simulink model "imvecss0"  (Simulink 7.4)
settings: Solver=ode45  StartTime=0  StopTime=20  MaxStep=5e-4  RelTol=1e-3

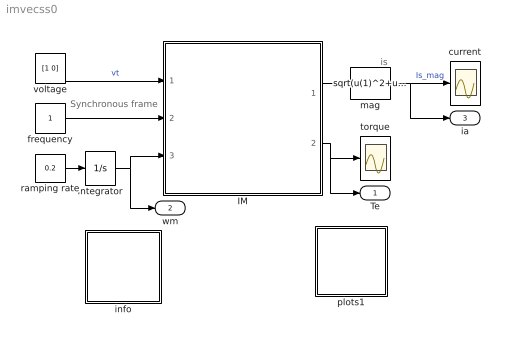
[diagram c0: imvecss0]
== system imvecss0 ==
  note: is
  note: Synchronous frame
  IM : Subsystem  mask(Inductionmachine){Rs=0.01, Rr=0.02, Lsl=0.10, Lrl=0.10, Lm=4.50, wo=2*pi*60}
      mask prompts: Rs "Stator resistance [pu]"; Rr "Rotor resistance [pu]"; Lsl "Stator leakage inductance [pu]"; Lrl "Rotor leakage inductance [pu]"; Lm "Magnetizing inductance [pu]"; wo "Base frequency [rad/s]"
      mask help: Induction motor subsystem model using state space formulation in an arbitrary reference frame k. Parameters are expressed in per unit.
  Integrator : Integrator  InitialCondition=-1  LimitOutput=on  UpperSaturationLimit=2  LowerSaturationLimit=-2
  current : Scope
  frequency : Constant  OutDataType=sfix(16)  OutScaling=2^0
  info : Subsystem
  mag : Fcn  Expr=sqrt(u(1)^2+u(2)^2)
  plots1 : Subsystem
  ramping rate : Constant  Value=0.2  OutDataType=sfix(16)  OutScaling=2^0
  torque : Scope
  voltage : Constant  Value=[1 0]  OutDataType=sfix(16)  OutScaling=2^0
  Te : Outport
  wm : Outport  Port=2
  ia : Outport  Port=3
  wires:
  frequency/1 -> IM/2(wk)
  voltage/1 -> IM/1(vs)  "vt"
  ramping rate/1 -> Integrator/1
  Integrator/1 -> IM/3(wm), wm/1
  mag/1 -> current/1, ia/1  "Is_mag"
  IM/1(is) -> mag/1
  IM/2(Te) -> torque/1, Te/1

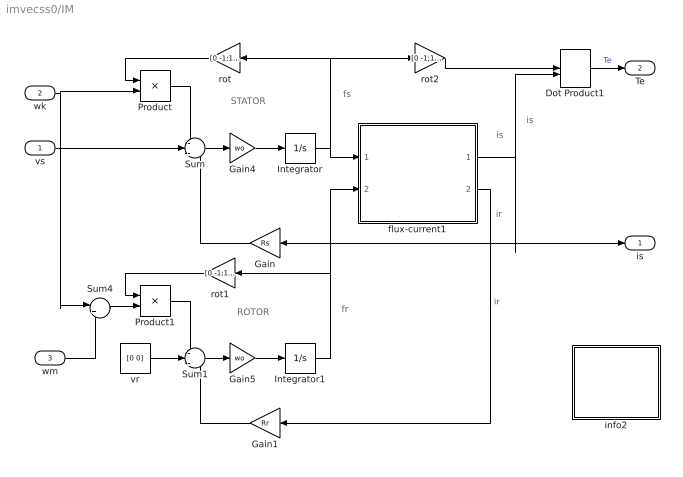
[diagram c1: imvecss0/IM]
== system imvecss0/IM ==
  note: ROTOR
  note: STATOR
  note: fs
  note: fr
  note: is
  note: is
  note: ir
  vs : Inport  OutDataType=sfix(16)  OutScaling=2^0
  wk : Inport  Port=2  OutDataType=sfix(16)  OutScaling=2^0
  wm : Inport  Port=3  OutDataType=sfix(16)  OutScaling=2^0
  Dot Product1 : DotProduct  OutDataType=fixdt(1, 16)  OutScaling=2^-10
  Gain : Gain  Gain=Rs  ParameterDataType=sfix(16)  ParameterScaling=2^0  OutDataType=sfix(16)  OutScaling=2^0
  Gain1 : Gain  Gain=Rr  ParameterDataType=sfix(16)  ParameterScaling=2^0  OutDataType=sfix(16)  OutScaling=2^0
  Gain4 : Gain  Gain=wo  ParameterDataType=sfix(16)  ParameterScaling=2^0  OutDataType=sfix(16)  OutScaling=2^0
  Gain5 : Gain  Gain=wo  ParameterDataType=sfix(16)  ParameterScaling=2^0  OutDataType=sfix(16)  OutScaling=2^0
  Integrator : Integrator  InitialCondition=[0 0]
  Integrator1 : Integrator  InitialCondition=[0 0]
  Product : Product  OutDataType=sfix(16)  OutScaling=2^0
  Product1 : Product  OutDataType=sfix(16)  OutScaling=2^0
  Sum : Sum  Inputs=-+-  OutDataType=sfix(16)  OutScaling=2^0
  Sum1 : Sum  Inputs=-+-  OutDataType=sfix(16)  OutScaling=2^0
  Sum4 : Sum  Inputs=|+-  OutDataType=sfix(16)  OutScaling=2^0
  flux-current1 : Subsystem
  info2 : Subsystem
  rot : Gain  Gain=[0 -1;1 0]  Multiplication=Matrix(K*u)  ParameterDataType=sfix(16)  ParameterScaling=2^0  OutDataType=sfix(16)  OutScaling=2^0
  rot1 : Gain  Gain=[0 -1;1 0]  Multiplication=Matrix(K*u)  ParameterDataType=sfix(16)  ParameterScaling=2^0  OutDataType=sfix(16)  OutScaling=2^0
  rot2 : Gain  Gain=[0 -1;1 0]  Multiplication=Matrix(K*u)  ParameterDataType=sfix(16)  ParameterScaling=2^0  OutDataType=sfix(16)  OutScaling=2^0
  vr : Constant  Value=[0 0]  OutDataType=sfix(16)  OutScaling=2^0
  is : Outport
  Te : Outport  Port=2
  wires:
  Gain/1 -> Sum/3
  vr/1 -> Sum1/2
  Gain1/1 -> Sum1/3
  flux-current1/2(ir) -> Gain1/1  "ir"
  Integrator/1 -> flux-current1/1(fs), rot/1, rot2/1
  Integrator1/1 -> rot1/1, flux-current1/2(fr)
  Product1/1 -> Sum1/1
  rot1/1 -> Product1/1
  Product/1 -> Sum/1
  rot/1 -> Product/1
  rot2/1 -> Dot Product1/1
  Sum4/1 -> Product1/2
  Sum/1 -> Gain4/1
  Gain4/1 -> Integrator/1
  Sum1/1 -> Gain5/1
  Gain5/1 -> Integrator1/1
  flux-current1/1(is) -> Gain/1, is/1, Dot Product1/2
  Dot Product1/1 -> Te/1  "Te"
  vs/1 -> Sum/2
  wk/1 -> Product/2, Sum4/1
  wm/1 -> Sum4/2

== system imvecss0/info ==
  note: Steady-state characteristics of an induction machine
  note: This demonstration illustrates how to obtain the steady-state characteristics of an induction motor using the dynamic model representation. Double click to view the torque- and current-speed curves. To modify the machine parameters, double click the induction motor block.

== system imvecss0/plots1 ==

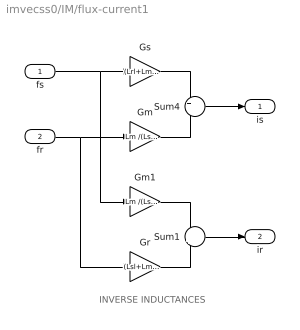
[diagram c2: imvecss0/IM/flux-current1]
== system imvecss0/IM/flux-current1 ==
  note: INVERSE INDUCTANCES
  fs : Inport  OutDataType=sfix(16)  OutScaling=2^0
  fr : Inport  Port=2  OutDataType=sfix(16)  OutScaling=2^0
  Gm : Gain  Gain=Lm /(Lsl*Lrl+Lsl*Lm+Lrl*Lm)  ParameterDataType=sfix(16)  ParameterScaling=2^0  OutDataType=sfix(16)  OutScaling=2^0
  Gm1 : Gain  Gain=Lm /(Lsl*Lrl+Lsl*Lm+Lrl*Lm)  ParameterDataType=sfix(16)  ParameterScaling=2^0  OutDataType=sfix(16)  OutScaling=2^0
  Gr : Gain  Gain=(Lsl+Lm )/(Lsl*Lrl+Lsl*Lm+Lrl*Lm)  ParameterDataType=sfix(16)  ParameterScaling=2^0  OutDataType=sfix(16)  OutScaling=2^0
  Gs : Gain  Gain=(Lrl+Lm) /(Lsl*Lrl+Lsl*Lm+Lrl*Lm)  ParameterDataType=sfix(16)  ParameterScaling=2^0  OutDataType=sfix(16)  OutScaling=2^0
  Sum1 : Sum  Inputs=-+  OutDataType=sfix(16)  OutScaling=2^0
  Sum4 : Sum  Inputs=+-  OutDataType=sfix(16)  OutScaling=2^0
  is : Outport
  ir : Outport  Port=2
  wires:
  fs/1 -> Gs/1, Gm1/1
  Gs/1 -> Sum4/1
  fr/1 -> Gm/1, Gr/1
  Gm/1 -> Sum4/2
  Sum4/1 -> is/1
  Gm1/1 -> Sum1/1
  Gr/1 -> Sum1/2
  Sum1/1 -> ir/1

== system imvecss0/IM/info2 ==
  note: Synchronous machine transients under shortcircuit
  note: This demonstration illustrates the dynamics of a synchronous generator, initially at no load, following a three-phase short circuit at the terminals.
